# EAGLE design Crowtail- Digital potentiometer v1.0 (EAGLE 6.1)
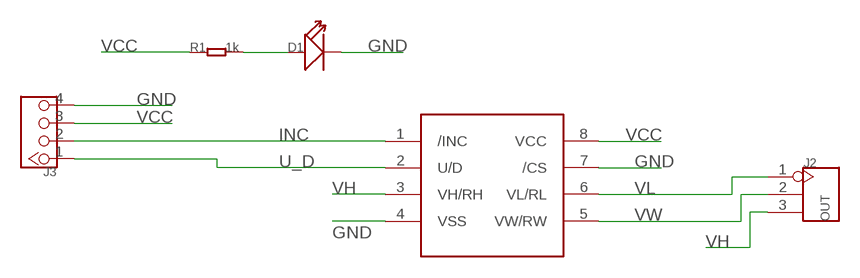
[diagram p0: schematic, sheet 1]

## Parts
D1  LED'0603'  [LED-0603]
J2  OUT  HEADER-3P-2.54  [3P-2.54]
J3  TWIG-4P-2.0-2.0  [4P-2.0]
R1  1k  R-0603  [0603]
U1  X9C103S  [SOP8]

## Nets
GND: D1.- J3.4 U1.4(VSS) U1.7(/CS)
INC: J3.2 U1.1(/INC)
N$5: D1.+ R1.2
U_D: J3.1 U1.2(U/D)
VCC: J3.3 R1.1 U1.8(VCC)
VH: J2.3 U1.3(VH/RH)
VL: J2.1 U1.6(VL/RL)
VW: J2.2 U1.5(VW/RW)

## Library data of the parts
D1 = Discrete:LED*
J2 = Connector:HEADER-3P
J3 = Connector:TWIG-4P-2.0
R1 = Discrete:R*
U1 = IC:X9C103S

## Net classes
0 default: width 0.203 mm, drill 0.305 mm, clearance 0.152 mm

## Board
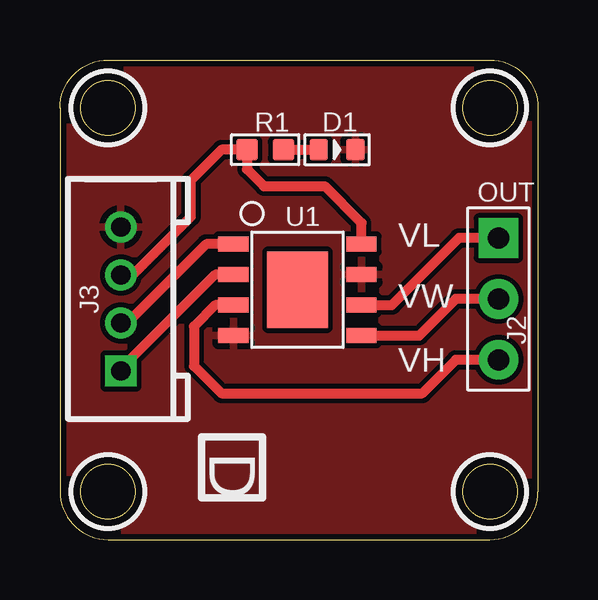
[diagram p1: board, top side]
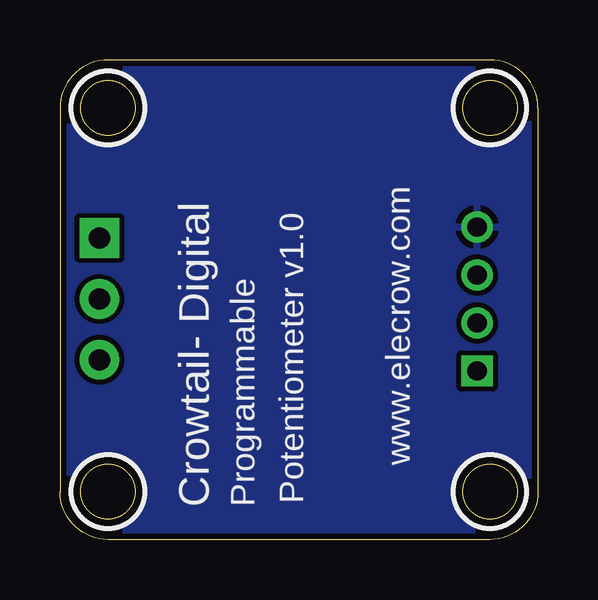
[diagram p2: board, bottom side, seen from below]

Size 19.93 x 20 mm. Coordinates in mm from the lower left corner, seen from the top.
Outline: 0,18 0,2 arc90 2,0 17.93,0 arc90 19.93,2 19.93,18 arc90 17.93,20 2,20 arc90 0,18
Outline: circle at 2,18 radius 1.14
Outline: circle at 2,18 radius 1.14
Outline: circle at 2,2 radius 1.14
Outline: circle at 17.93,18 radius 1.14
Outline: circle at 17.93,18 radius 1.14
Outline: circle at 17.93,2 radius 1.14
Outline: circle at 17.93,2 radius 1.14
Copper layers (1*16): Top 0.035mm / dielectric 1.5mm / Bottom 0.035mm
Design rules: minimum track width 10mil, minimum drill 10mil, track to track 8mil, track to pad 8mil, pad to pad 8mil, via to via 8mil, smd to smd 8mil, copper to edge 10mil, drill to drill 8mil, minimum pad ring 10mil, minimum via ring 8mil, stop-mask expansion 4mil, vias tented up to drill 100mil, thermal gap 10mil
tRestrict: area 0.5,16.5 to 3.5,19.5; area 0.5,0.5 to 3.5,3.5; area 16.4,16.5 to 19.5,19.5; area 16.4,0.5 to 19.5,3.5
bRestrict: area 0.5,16.5 to 3.5,19.5; area 0.5,0.5 to 3.5,3.5; area 16.4,16.5 to 19.5,19.5; area 16.4,0.5 to 19.5,3.5

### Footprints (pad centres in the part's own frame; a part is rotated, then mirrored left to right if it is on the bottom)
LED-0603 = smd 0.762 x 0.889: + -0.762,0; - 0.762,0
3P-2.54 = drill 0.889 pad 1.651 square: 1 0,2.54 | drill 0.889 pad 1.651: 2 0,0; 3 0,-2.54
4P-2.0 = drill 0.8 pad 1.27 square: 1 -3,0 | drill 0.8 pad 1.27: 2 -1,0; 3 1,0; 4 3,0
0603 = smd 0.889 x 0.889: 1 -0.762,0; 2 0.762,0
SOP8 = smd 0.635 x 1.27: 1 -1.905,-2.667; 2 -0.635,-2.667; 3 0.635,-2.667; 4 1.905,-2.667; 5 1.905,2.667; 6 0.635,2.667; 7 -0.635,2.667; 8 -1.905,2.667 | smd 3.175 x 2.54: HEAT 0,0

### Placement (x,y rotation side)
D1  11.56,16.26 0 top
J2  18.29,10.03 0 top
J3  2.54,10.03 90 top
R1  8.56,16.26 0 top
U1  9.91,10.41 270 top

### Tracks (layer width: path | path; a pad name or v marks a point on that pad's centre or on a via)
GND
  pour Top: -0.76,20.83 20.83,20.83 20.83,-0.64 -0.76,-0.64
  pour Bottom: -0.64,20.7 20.7,20.7 20.7,-0.51 -0.64,-0.51
INC
  Top 0.406: J3.2 2.81,9.03 6.1,12.32 U1.1
N$5
  Top 0.406: R1.2 D1.+
U_D
  Top 0.406: 7.22,11.03 U1.2 6.48,11.05 2.54,7.11 J3.1
VCC
  Top 0.406: U1.8 12.57,13.21 11.05,14.73 8.51,14.73 7.79,15.45 R1.1 6.74,16.26 5.46,14.99 5.46,13.46 3.03,11.03 J3.3
VH
  Top 0.406: U1.3 6.48,9.78 5.59,8.89 5.59,7.24 6.73,6.1 15.11,6.1 16.51,7.49 J2.3
VL
  Top 0.406: U1.6 13.84,9.78 16.64,12.57 J2.1
VW
  Top 0.406: U1.5 14.99,8.51 16.51,10.03 J2.2

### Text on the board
tPlace: D
bPlace: www.elecrow.com | Potentiometer v1.0 | Programmable | Crowtail- Digital
tNames: OUT | VL | VW | VH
